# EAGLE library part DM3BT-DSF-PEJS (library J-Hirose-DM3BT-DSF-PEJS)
HIROSE - microSD Card socket - Reverse on-Board - Push / Push
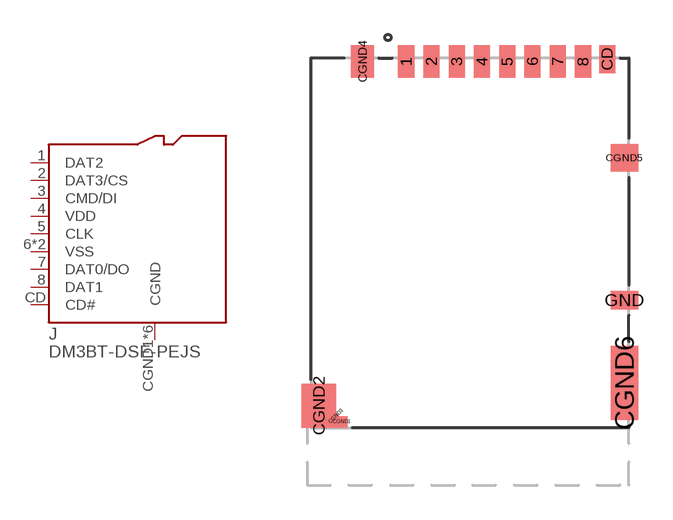
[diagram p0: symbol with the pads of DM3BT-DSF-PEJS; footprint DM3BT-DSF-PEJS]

Designator prefix J

## DM3BT-DSF-PEJS  [DM3BT-DSF-PEJS]
1  DAT2
2  DAT3/CS
3  CMD/DI
4  VDD
5  CLK
6  VSS
7  DAT0/DO
8  DAT1
CD  CD#
CGND1  CGND
CGND2  CGND
CGND3  CGND
CGND4  CGND
CGND5  CGND
CGND6  CGND
GND  VSS

## Footprint DM3BT-DSF-PEJS (pad centres in mm)
smd 0.7 x 1.4: 1 -3.2,15.95; 2 -2.1,15.95; 3 -1,15.95; 4 0.1,15.95; 5 1.2,15.95; 6 2.3,15.95; 7 3.4,15.95; 8 4.5,15.95
smd 0.7 x 1.2: CD 5.55,16.05
smd 0.5 x 0.5: CGND1 -6,0.25
smd 1.5 x 1.9: CGND2 -7,0.95
smd 0.21 x 0.21 rotated 45: CGND3 -6.25,0.5
smd 1 x 1.4: CGND4 -5.1,15.95
smd 1.2 x 1.2: CGND5 6.3,11.75
smd 1.2 x 3.2: CGND6 6.3,1.95
smd 1.2 x 0.8: GND 6.3,5.55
